(* Logix 5000 AddOnInstructionDefinition export B256_StoC_LE; software revision 30.00 *)

ADD_ON_INSTRUCTION D_SHR   (* revision 1.0, vendor Ken Fischer, NSWCPD, C512 *)
// DINT bit shift right of the 32-bit argument Inp_A by Inp_B bits with paddding by zeros on the right
// Revision note:
// Rev1.0: TBD - Initial Release
VAR_IN_OUT
   Inp_A : DINT; {required}   // 64-bit Integer to be right circular rotated
END_VAR
VAR_INPUT
   Inp_B : INT; {required}   // Number of bits to shift
END_VAR
VAR_IN_OUT
   Out : DINT; {required}   // Result
END_VAR
VAR
   BSR_Cntrl : CONTROL := (LEN := 32);
   ONS : BOOL;
   Source_Bit : BOOL;
   Wrk_InpA : DINT[2];
END_VAR

ROUTINE Logic   (* ladder *)
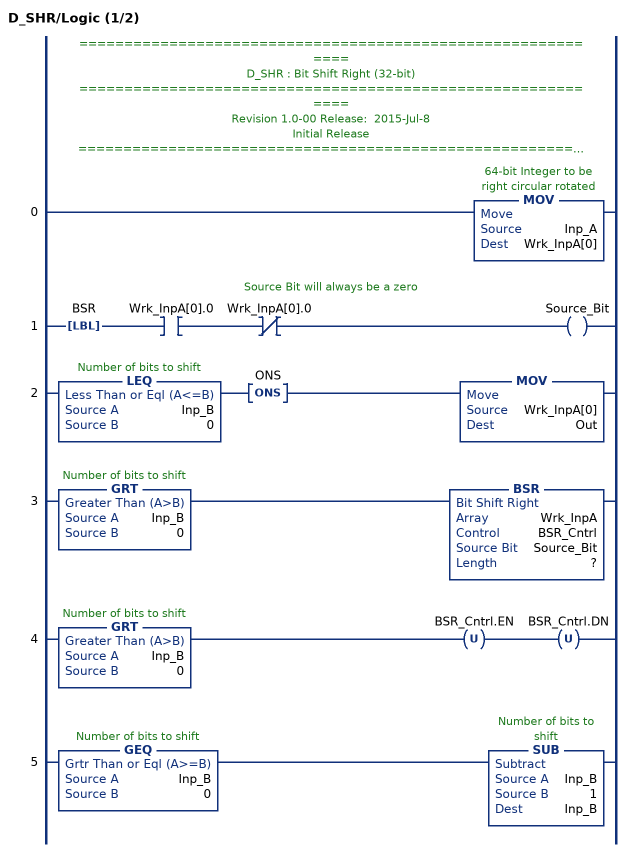
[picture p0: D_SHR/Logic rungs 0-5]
   // ============================================================
   // D_SHR : Bit Shift Right (32-bit)
   // ============================================================
   // Revision 1.0-00 Release:  2015-Jul-8
   // Initial Release
   // ============================================================
   // Performs a right bit shift of the 32-bit argument Inp_A by the
   // number of bits defined in the 16-bit argument Inp_B, with padding by zeros.
   0: MOV(Inp_A,Wrk_InpA[0]);
   // Source Bit will always be a zero
   1: LBL(BSR)XIC(Wrk_InpA[0].0)XIO(Wrk_InpA[0].0)OTE(Source_Bit);
   2: LEQ(Inp_B,0)ONS(ONS)MOV(Wrk_InpA[0],Out);
   3: GRT(Inp_B,0)BSR(Wrk_InpA,BSR_Cntrl,Source_Bit,?);
   4: GRT(Inp_B,0)OTU(BSR_Cntrl.EN)OTU(BSR_Cntrl.DN);
   5: GEQ(Inp_B,0)SUB(Inp_B,1,Inp_B);
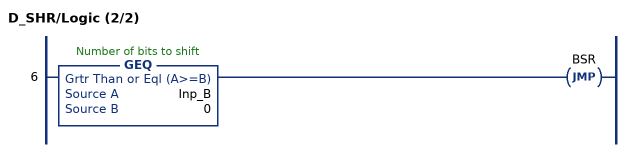
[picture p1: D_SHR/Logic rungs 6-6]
   6: GEQ(Inp_B,0)JMP(BSR);
END_ROUTINE
END_ADD_ON_INSTRUCTION

ADD_ON_INSTRUCTION D_SHL   (* revision 1.0, vendor Ken Fischer, NSWCPD, C512 *)
// DINT bit shift left of the 32-bit argument Inp_A by Inp_B bits with paddding by zeros on the right
// Revision note:
// Rev1.0: TBD - Initial Release
VAR_IN_OUT
   Inp_A : DINT; {required}   // 64-bit Integer to be right circular rotated
END_VAR
VAR_INPUT
   Inp_B : INT; {required}   // Number of bits to shift
END_VAR
VAR_IN_OUT
   Out : DINT; {required}   // Result
END_VAR
VAR
   Wrk_InpA : DINT[2];
   Source_Bit : BOOL;
   ONS : BOOL;
   BSL_Cntrl : CONTROL := (LEN := 32);
END_VAR

ROUTINE Logic   (* ladder *)
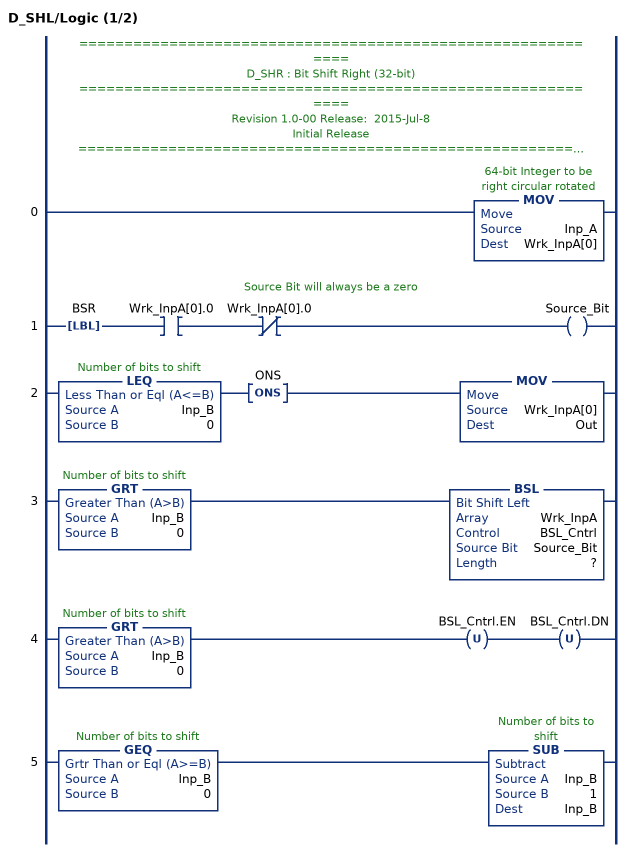
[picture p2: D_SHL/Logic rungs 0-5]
   // ============================================================
   // D_SHR : Bit Shift Right (32-bit)
   // ============================================================
   // Revision 1.0-00 Release:  2015-Jul-8
   // Initial Release
   // ============================================================
   // Performs a left bit shift of the 32-bit argument Inp_A by the
   // number of bits defined in the 16-bit argument Inp_B, with padding by zeros.
   0: MOV(Inp_A,Wrk_InpA[0]);
   // Source Bit will always be a zero
   1: LBL(BSR)XIC(Wrk_InpA[0].0)XIO(Wrk_InpA[0].0)OTE(Source_Bit);
   2: LEQ(Inp_B,0)ONS(ONS)MOV(Wrk_InpA[0],Out);
   3: GRT(Inp_B,0)BSL(Wrk_InpA,BSL_Cntrl,Source_Bit,?);
   4: GRT(Inp_B,0)OTU(BSL_Cntrl.EN)OTU(BSL_Cntrl.DN);
   5: GEQ(Inp_B,0)SUB(Inp_B,1,Inp_B);
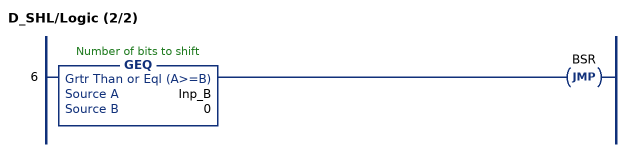
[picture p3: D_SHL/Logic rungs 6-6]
   6: GEQ(Inp_B,0)JMP(BSR);
END_ROUTINE
END_ADD_ON_INSTRUCTION

ADD_ON_INSTRUCTION B256_CtoE   (* revision 1.0 20170916, vendor Kenneth A. Fischer *)
// Convert 256-bit value using 22 12-bit pieces into 256-bit value using 32 8-bit pieces
// Revision note:
// Rev1.0: 20170916 - Initial Release
VAR_IN_OUT
   Inp_C : DINT[22]; {required}
   Out_E : DINT[32]; {required}
END_VAR
VAR
   i : INT;
   j : INT;
   TEMP1 : DINT;
   TEMP2 : DINT;
   D_SHL : D_SHL;
   D_SHR : D_SHR;
END_VAR

ROUTINE Logic   (* ladder *)
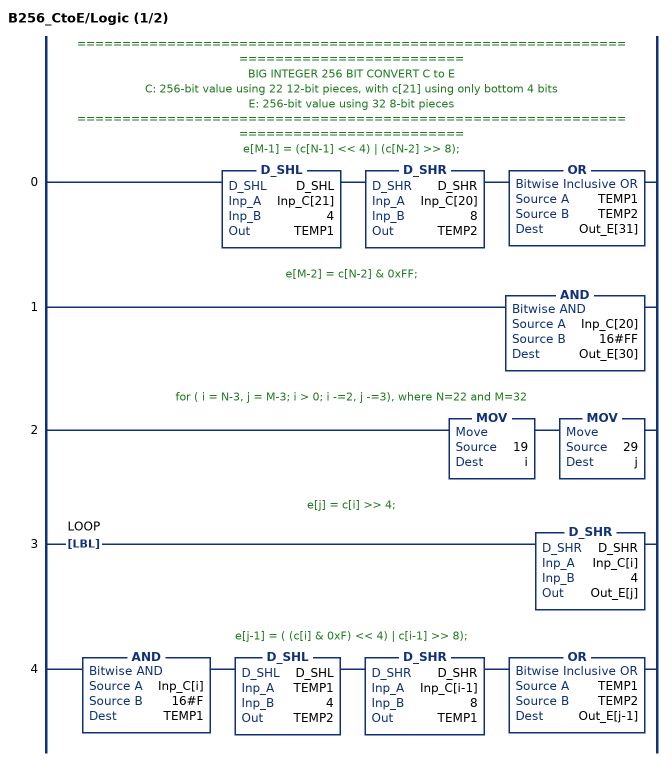
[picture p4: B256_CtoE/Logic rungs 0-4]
   // ======================================================================================
   // BIG INTEGER 256 BIT CONVERT C to E
   // C: 256-bit value using 22 12-bit pieces, with c[21] using only bottom 4 bits
   // E: 256-bit value using 32 8-bit pieces
   // ======================================================================================
   // e[M-1] = (c[N-1] << 4) | (c[N-2] >> 8);
   0: D_SHL(D_SHL,Inp_C[21],4,TEMP1)D_SHR(D_SHR,Inp_C[20],8,TEMP2)OR(TEMP1,TEMP2,Out_E[31]);
   // e[M-2] = c[N-2] & 0xFF;
   1: AND(Inp_C[20],16#FF,Out_E[30]);
   // for ( i = N-3, j = M-3; i > 0; i -=2, j -=3), where N=22 and M=32
   2: MOV(19,i)MOV(29,j);
   // e[j] = c[i] >> 4;
   3: LBL(LOOP)D_SHR(D_SHR,Inp_C[i],4,Out_E[j]);
   // e[j-1] = ( (c[i] & 0xF) << 4) | c[i-1] >> 8);
   4: AND(Inp_C[i],16#F,TEMP1)D_SHL(D_SHL,TEMP1,4,TEMP2)D_SHR(D_SHR,Inp_C[i-1],8,TEMP1)OR(TEMP1,TEMP2,Out_E[j-1]);
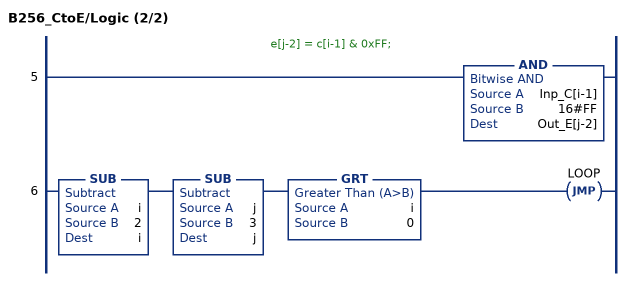
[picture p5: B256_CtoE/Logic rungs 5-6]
   // e[j-2] = c[i-1] & 0xFF;
   5: AND(Inp_C[i-1],16#FF,Out_E[j-2]);
   6: SUB(i,2,i)SUB(j,3,j)GRT(i,0)JMP(LOOP);
END_ROUTINE
END_ADD_ON_INSTRUCTION

ADD_ON_INSTRUCTION B256_EtoC   (* revision 1.0 20170916, vendor Kenneth A. Fischer *)
// Convert 256-bit value using 32 8-bit pieces into 256-bit value using 22 12-bit pieces
// Revision note:
// Rev1.0: 20170916 - Initial Release
VAR_IN_OUT
   Inp_E : DINT[32]; {required}
   Out_C : DINT[22]; {required}
END_VAR
VAR
   i : INT;
   j : INT;
   TEMP1 : DINT;
   TEMP2 : DINT;
   D_SHL : D_SHL;
   D_SHR : D_SHR;
END_VAR

ROUTINE Logic   (* ladder *)
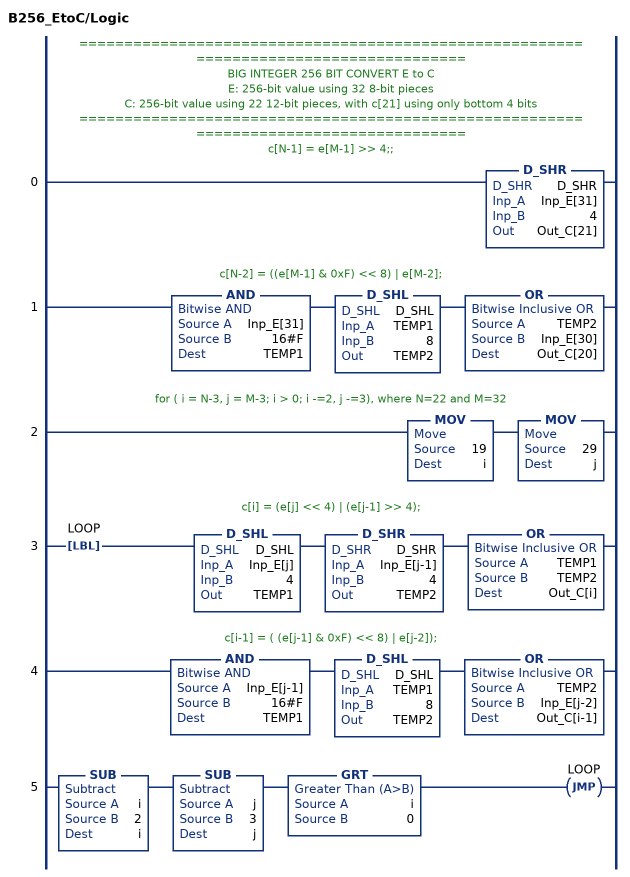
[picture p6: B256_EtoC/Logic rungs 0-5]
   // ======================================================================================
   // BIG INTEGER 256 BIT CONVERT E to C
   // E: 256-bit value using 32 8-bit pieces
   // C: 256-bit value using 22 12-bit pieces, with c[21] using only bottom 4 bits
   // ======================================================================================
   // c[N-1] = e[M-1] >> 4;;
   0: D_SHR(D_SHR,Inp_E[31],4,Out_C[21]);
   // c[N-2] = ((e[M-1] & 0xF) << 8) | e[M-2];
   1: AND(Inp_E[31],16#F,TEMP1)D_SHL(D_SHL,TEMP1,8,TEMP2)OR(TEMP2,Inp_E[30],Out_C[20]);
   // for ( i = N-3, j = M-3; i > 0; i -=2, j -=3), where N=22 and M=32
   2: MOV(19,i)MOV(29,j);
   // c[i] = (e[j] << 4) | (e[j-1] >> 4);
   3: LBL(LOOP)D_SHL(D_SHL,Inp_E[j],4,TEMP1)D_SHR(D_SHR,Inp_E[j-1],4,TEMP2)OR(TEMP1,TEMP2,Out_C[i]);
   // c[i-1] = ( (e[j-1] & 0xF) << 8) | e[j-2]);
   4: AND(Inp_E[j-1],16#F,TEMP1)D_SHL(D_SHL,TEMP1,8,TEMP2)OR(TEMP2,Inp_E[j-2],Out_C[i-1]);
   5: SUB(i,2,i)SUB(j,3,j)GRT(i,0)JMP(LOOP);
END_ROUTINE
END_ADD_ON_INSTRUCTION

ADD_ON_INSTRUCTION B256_StoC_LE   (* revision 1.0 20170916, vendor Kenneth A. Fischer *)
// Convert 256-bit value using 64 hex string characters into 256-bit value using 22 12-bit pieces
// Little Endian
// Revision note:
// Rev1.0: 20170916 - Initial Release
VAR_IN_OUT
   Temp_E : DINT[32]; {required}
   Inp_S : STRING; {required}
   Out_C : DINT[22]; {required}
END_VAR
VAR
   byte : DINT[3];
   D_SHL : D_SHL;
   i : INT;
   j : INT;
   k : DINT;
   temp : DINT;
   B256_CtoE : B256_CtoE;
   E : DINT[32];
   B256_EtoC : B256_EtoC;
END_VAR

ROUTINE Logic   (* ladder *)
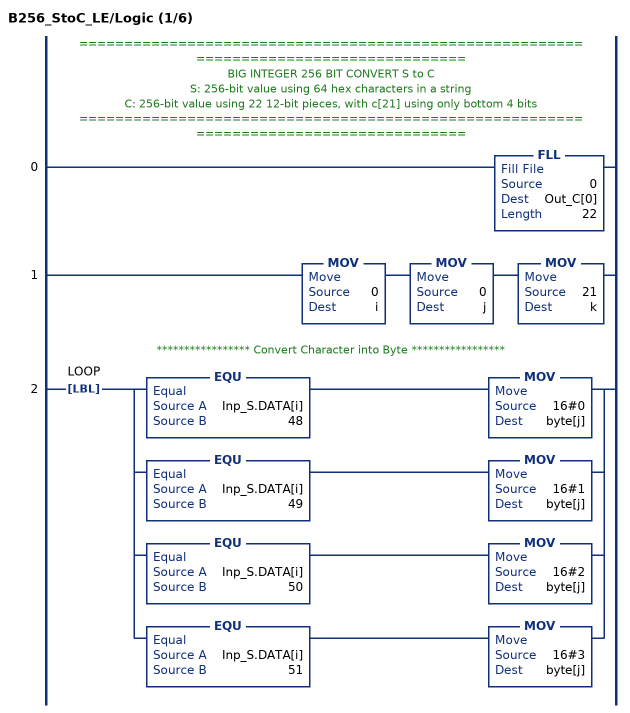
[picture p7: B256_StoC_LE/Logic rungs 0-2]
   // ======================================================================================
   // BIG INTEGER 256 BIT CONVERT S to C
   // S: 256-bit value using 64 hex characters in a string
   // C: 256-bit value using 22 12-bit pieces, with c[21] using only bottom 4 bits
   // ======================================================================================
   0: FLL(0,Out_C[0],22);
   1: MOV(0,i)MOV(0,j)MOV(21,k);
   // ***************** Convert Character into Byte *****************
   2: LBL(LOOP)[EQU(Inp_S.DATA[i],48) MOV(16#0,byte[j]) ,EQU(Inp_S.DATA[i],49) MOV(16#1,byte[j]) ,EQU(Inp_S.DATA[i],50) MOV(16#2,byte[j]) ,EQU(Inp_S.DATA[i],51) MOV(16#3,byte[j]) ];
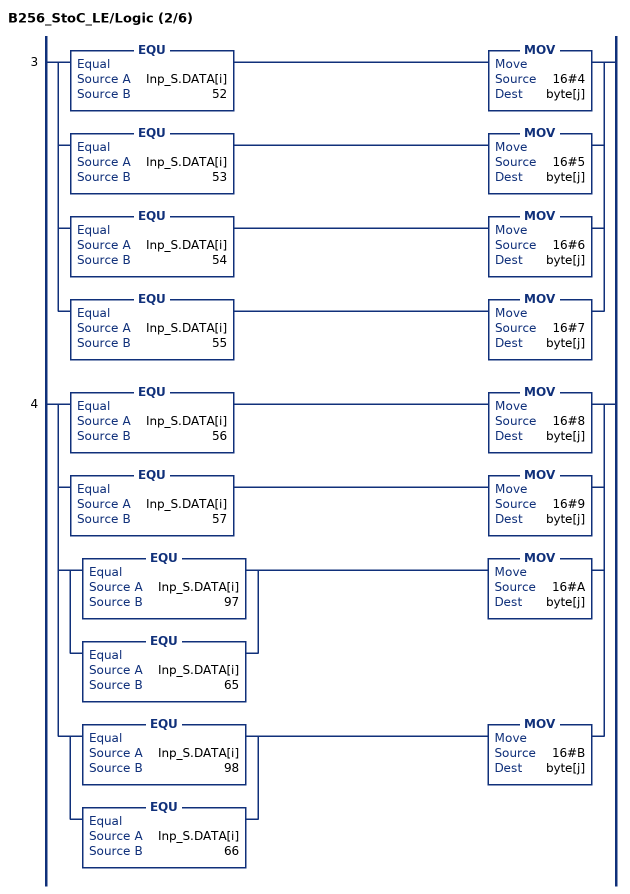
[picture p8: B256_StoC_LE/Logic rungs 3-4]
   3: [EQU(Inp_S.DATA[i],52) MOV(16#4,byte[j]) ,EQU(Inp_S.DATA[i],53) MOV(16#5,byte[j]) ,EQU(Inp_S.DATA[i],54) MOV(16#6,byte[j]) ,EQU(Inp_S.DATA[i],55) MOV(16#7,byte[j]) ];
   4: [EQU(Inp_S.DATA[i],56) MOV(16#8,byte[j]) ,EQU(Inp_S.DATA[i],57) MOV(16#9,byte[j]) ,[EQU(Inp_S.DATA[i],97) ,EQU(Inp_S.DATA[i],65) ] MOV(16#A,byte[j]) ,[EQU(Inp_S.DATA[i],98) ,EQU(Inp_S.DATA[i],66) ] MOV(16#B,byte[j]) ];
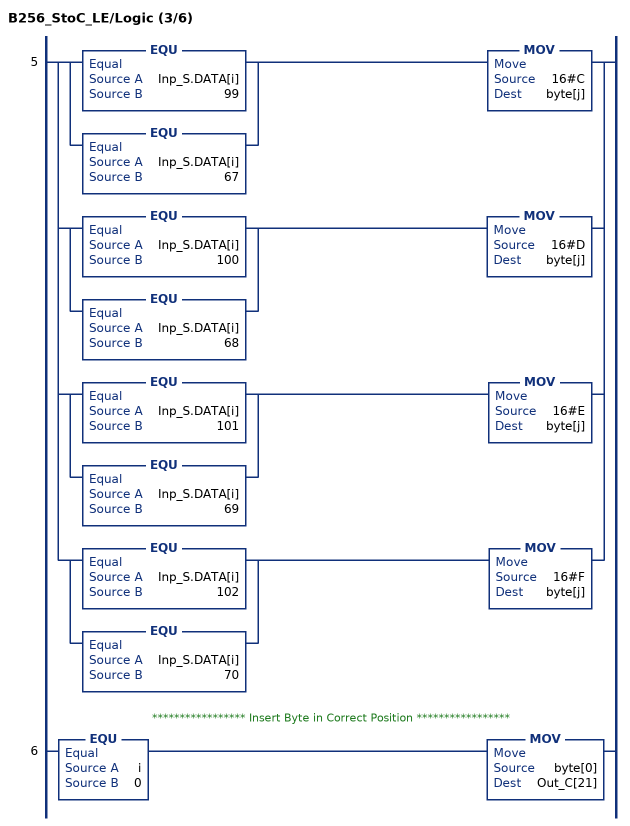
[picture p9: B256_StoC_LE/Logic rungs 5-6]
   5: [[EQU(Inp_S.DATA[i],99) ,EQU(Inp_S.DATA[i],67) ] MOV(16#C,byte[j]) ,[EQU(Inp_S.DATA[i],100) ,EQU(Inp_S.DATA[i],68) ] MOV(16#D,byte[j]) ,[EQU(Inp_S.DATA[i],101) ,EQU(Inp_S.DATA[i],69) ] MOV(16#E,byte[j]) ,[EQU(Inp_S.DATA[i],102) ,EQU(Inp_S.DATA[i],70) ] MOV(16#F,byte[j]) ];
   // ***************** Insert Byte in Correct Position *****************
   6: EQU(i,0)MOV(byte[0],Out_C[21]);
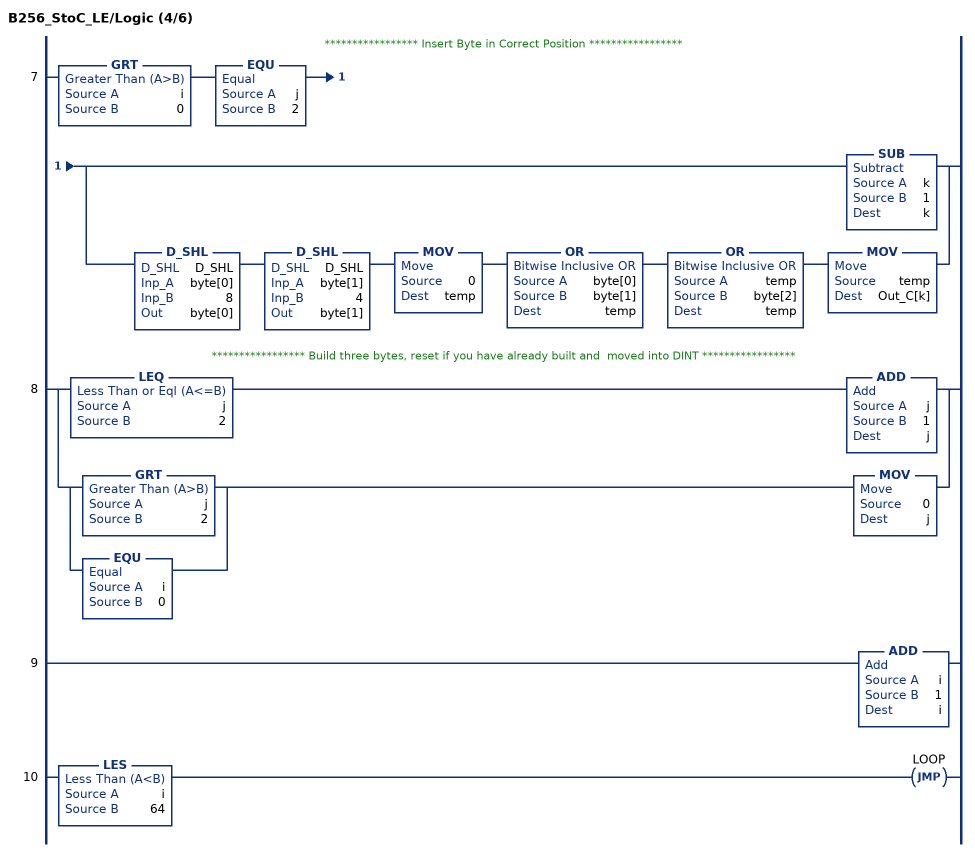
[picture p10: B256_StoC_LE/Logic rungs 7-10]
   // ***************** Insert Byte in Correct Position *****************
   7: GRT(i,0)EQU(j,2)[SUB(k,1,k) ,D_SHL(D_SHL,byte[0],8,byte[0]) D_SHL(D_SHL,byte[1],4,byte[1]) MOV(0,temp) OR(byte[0],byte[1],temp) OR(temp,byte[2],temp) MOV(temp,Out_C[k]) ];
   // ***************** Build three bytes, reset if you have already built and  moved into DINT *****************
   8: [LEQ(j,2) ADD(j,1,j) ,[GRT(j,2) ,EQU(i,0) ] MOV(0,j) ];
   9: ADD(i,1,i);
   10: LES(i,64)JMP(LOOP);
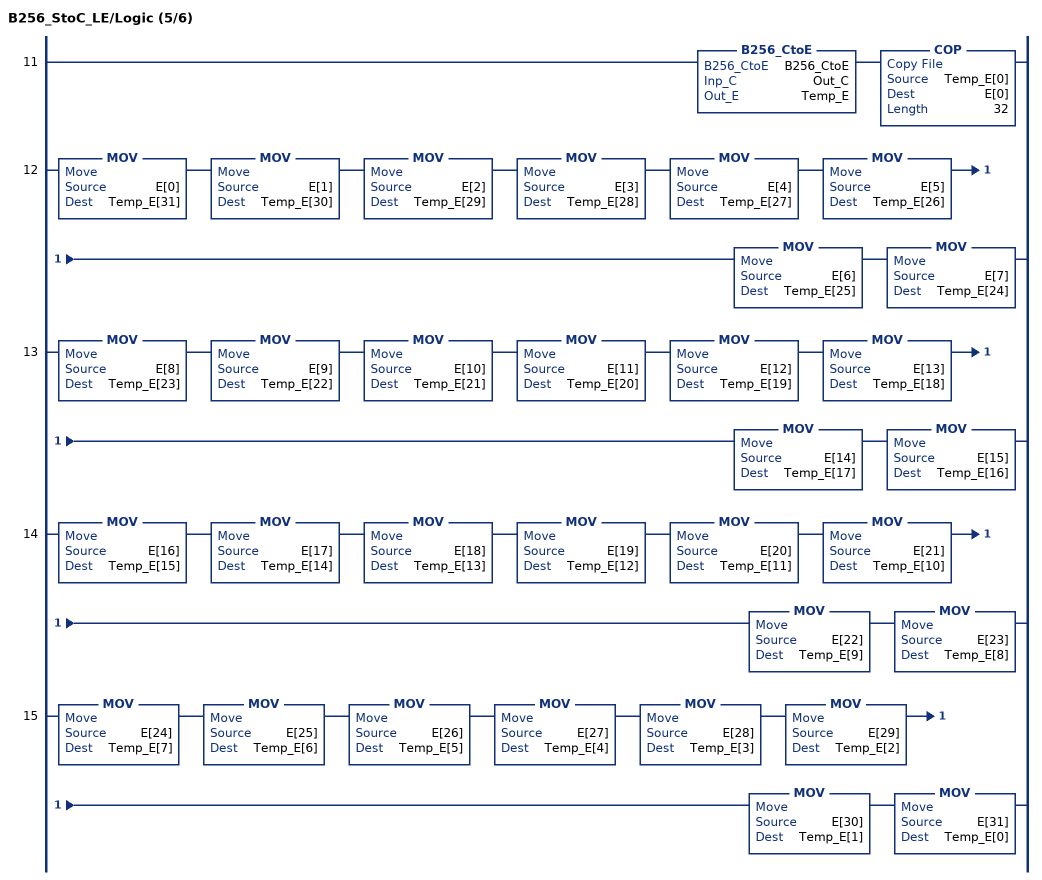
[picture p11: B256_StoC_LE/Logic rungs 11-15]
   11: B256_CtoE(B256_CtoE,Out_C,Temp_E)COP(Temp_E[0],E[0],32);
   12: MOV(E[0],Temp_E[31])MOV(E[1],Temp_E[30])MOV(E[2],Temp_E[29])MOV(E[3],Temp_E[28])MOV(E[4],Temp_E[27])MOV(E[5],Temp_E[26])MOV(E[6],Temp_E[25])MOV(E[7],Temp_E[24]);
   13: MOV(E[8],Temp_E[23])MOV(E[9],Temp_E[22])MOV(E[10],Temp_E[21])MOV(E[11],Temp_E[20])MOV(E[12],Temp_E[19])MOV(E[13],Temp_E[18])MOV(E[14],Temp_E[17])MOV(E[15],Temp_E[16]);
   14: MOV(E[16],Temp_E[15])MOV(E[17],Temp_E[14])MOV(E[18],Temp_E[13])MOV(E[19],Temp_E[12])MOV(E[20],Temp_E[11])MOV(E[21],Temp_E[10])MOV(E[22],Temp_E[9])MOV(E[23],Temp_E[8]);
   15: MOV(E[24],Temp_E[7])MOV(E[25],Temp_E[6])MOV(E[26],Temp_E[5])MOV(E[27],Temp_E[4])MOV(E[28],Temp_E[3])MOV(E[29],Temp_E[2])MOV(E[30],Temp_E[1])MOV(E[31],Temp_E[0]);
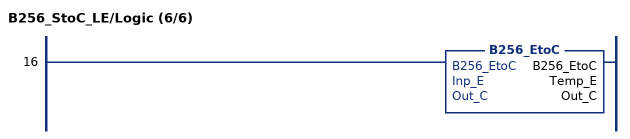
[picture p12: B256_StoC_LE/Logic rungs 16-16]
   16: B256_EtoC(B256_EtoC,Temp_E,Out_C);
END_ROUTINE
END_ADD_ON_INSTRUCTION
